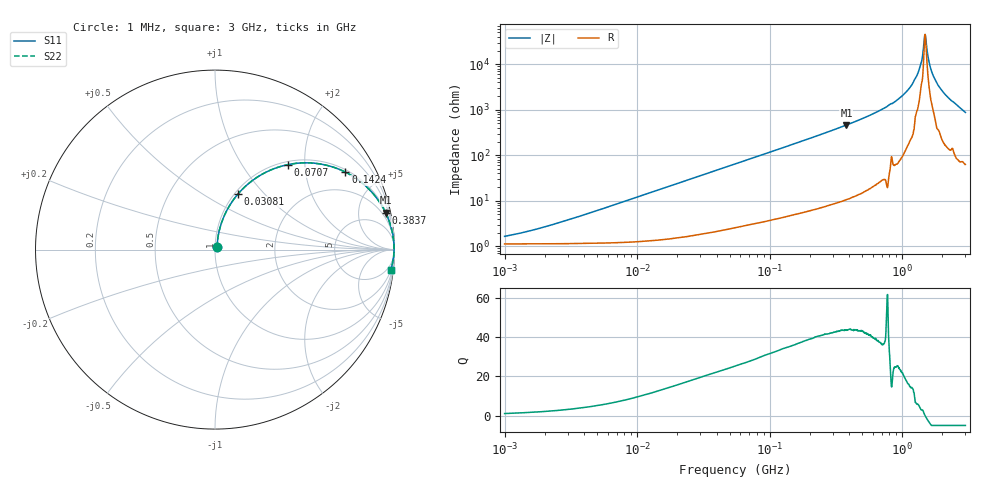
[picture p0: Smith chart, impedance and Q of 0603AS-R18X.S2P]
!s-Parameter Generated by FASTRON Sdn. Bhd.
!FASTRON P/N : 0603AS-R18X
!Keysight Technologies: E4991B_MY54100416_A.01.15
!Date created: Wed Sep 27 15:52:42 2023
!Version  : Rev01 Wed Sep 27 15:52:42 2023
!Data & Calibration Information:
!Freq	S11	S21	S12	S22
!PortZ  Port1:50+j0  Port2:50+j0
!When reading reference impedance value at option line is always used.
! Remarks : This data is being provided solely for informational purposes.
# Hz S dB R 50
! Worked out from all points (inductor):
!   1601 points, 1 MHz to 3 GHz, reference 50 ohm
!   read as one part in series: L = 191 nH near 2.86 MHz
!   highest Q = 43.7 at 379.8 MHz (marker M1), where L = 193 nH
!   self-resonance near 1.489 GHz
!   S11 on the Smith chart (normalised r, x): 1 MHz: 1.02, +0.02; 30.81 MHz: 1.04, +0.73; 70.7 MHz: 1.06, +1.65; 142.4 MHz: 1.09, +3.31; 383.7 MHz: 1.21, +9.32; 3 GHz: 2, -17
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1000000  -35.77 46.3  -0.10 -0.7  -0.10 -0.7  -35.77 46.3
3804036  -26.67 73.3  -0.11 -2.6  -0.11 -2.6  -26.67 73.3
1.447069e7  -15.50 75.8  -0.24 -9.6  -0.24 -9.6  -15.50 75.8
3.080651e7  -9.46 67.5  -0.68 -19.6  -0.68 -19.6  -9.46 67.5
5.477226e7  -5.51 55.7  -1.65 -32.0  -1.65 -32.0  -5.51 55.7
7.069584e7  -4.08 49.3  -2.40 -38.7  -2.40 -38.7  -4.08 49.3
1.424433e8  -1.46 30.7  -5.83 -57.7  -5.83 -57.7  -1.46 30.7
2.083556e8  -0.76 22.1  -8.47 -66.4  -8.47 -66.4  -0.76 22.1
3.798301e8  -0.24 12.2  -13.51 -76.5  -13.51 -76.5  -0.24 12.2
3.836505e8  -0.24 12.0  -13.61 -76.6  -13.61 -76.6  -0.24 12.0
7.925923e8  -0.05 4.5  -22.06 -84.0  -22.06 -84.0  -0.05 4.5
9.927591e8  -0.03 2.9  -25.97 -84.5  -25.97 -84.5  -0.03 2.9
1.182785e9  -0.02 1.6  -30.95 -84.4  -30.95 -84.4  -0.02 1.6
1.347129e9  -0.02 0.7  -37.92 -77.5  -37.92 -77.5  -0.02 0.7
1.388188e9  -0.03 0.5  -40.48 -71.1  -40.48 -71.1  -0.03 0.5
1.452135e9  -0.02 0.2  -48.13 -59.4  -48.13 -59.4  -0.02 0.2
1.496395e9  -0.02 -0.0  -52.80 13.5  -52.80 13.5  -0.02 -0.0
1.526649e9  -0.02 -0.2  -48.27 52.1  -48.27 52.1  -0.02 -0.2
1.653904e9  -0.02 -0.7  -37.51 77.4  -37.51 77.4  -0.02 -0.7
1.846379e9  -0.03 -1.6  -31.22 82.5  -31.22 82.5  -0.03 -1.6
2.23307e9  -0.05 -3.1  -25.28 82.5  -25.28 82.5  -0.05 -3.1
3e9  -0.13 -6.5  -18.93 79.4  -18.93 79.4  -0.13 -6.5
